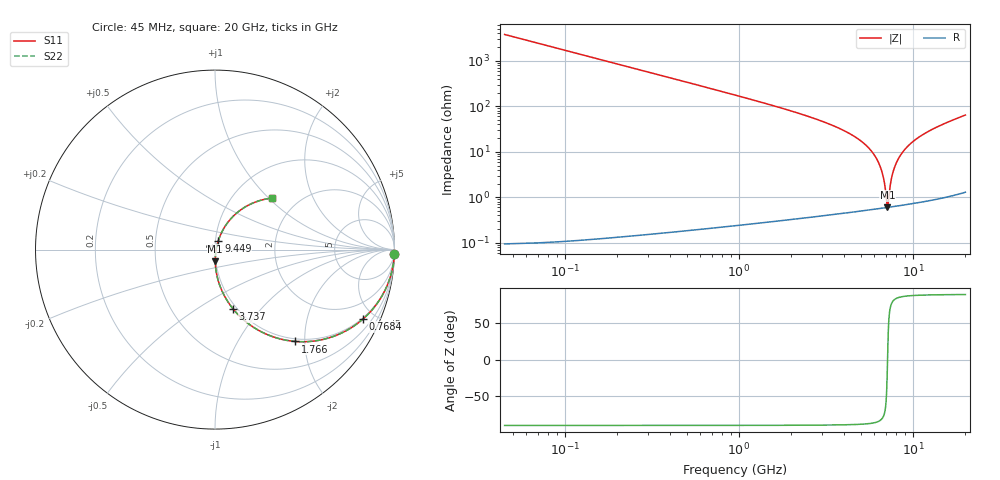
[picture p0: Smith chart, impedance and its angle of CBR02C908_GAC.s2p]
! S-parameter model data by Modelithics Inc.  support@modelithics.com 813-866-6335  Tampa FL USA
! S-Parameter data specifications:
! Substrate: 20-mil Rogers 4350B, substrate thickness, H=0.508mm, Dielectric constant, Er=3.75
! PCB Mounting Pad Footprint: Pad width, PadW=0.32mm , Pad length, PadL=0.37mm , Pad gap, PadG (edge-to-edge)=0.19mm , Reference planes=0.93mm apart
#  GHz  S  MA  R 50
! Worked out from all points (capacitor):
!   801 points, 45 MHz to 20 GHz, reference 50 ohm
!   read as one part in series: C = 929 fF near 144.8 MHz
!   lowest |Z| = 604 mohm at 7.129 GHz (marker M1)
!   series resonance near 7.139 GHz, so ESL is about 530 pH
!   S11 on the Smith chart (normalised r, x): 45 MHz: 1, -74; 768.4 MHz: 0.94, -4.29; 1.766 GHz: 0.95, -1.80; 3.737 GHz: 0.96, -0.72; 9.449 GHz: 1.03, +0.10; 20 GHz: 1.50, +1.05
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0.045  0.9997 -1.6  0.02626 88.4  0.02626 88.4  0.9997 -1.6
0.194662  0.9936 -6.7  0.113 83.3  0.113 83.3  0.9936 -6.7
0.319381  0.983 -10.9  0.1835 79.1  0.1835 79.1  0.983 -10.9
0.518931  0.9566 -17.5  0.2908 72.5  0.2908 72.5  0.9566 -17.5
0.768369  0.9108 -25.1  0.4119 64.8  0.4119 64.8  0.9108 -25.1
1.217356  0.8086 -37.2  0.5867 52.7  0.5867 52.7  0.8086 -37.2
1.766119  0.679 -48.9  0.7318 40.9  0.7318 40.9  0.679 -48.9
3.387462  0.3894 -70.1  0.9173 19.4  0.9173 19.4  0.3894 -70.1
3.736675  0.3446 -73.1  0.9347 16.2  0.9347 16.2  0.3446 -73.1
5.532625  0.1722 -84.2  0.9799 4.1  0.9799 4.1  0.1722 -84.2
6.704981  0.09132 -88.2  0.99 -1.8  0.99 -1.8  0.09132 -88.2
7.129025  0.0658 -88.6  0.9918 -3.7  0.9918 -3.7  0.0658 -88.6
7.802506  0.02851 -84.0  0.9932 -6.6  0.9932 -6.6  0.02851 -84.0
8.326325  0.006492 -13.8  0.9934 -8.7  0.9934 -8.7  0.006492 -13.8
8.4261  0.007877 25.2  0.9933 -9.1  0.9933 -9.1  0.007877 25.2
8.850144  0.02605 64.4  0.9928 -10.7  0.9928 -10.7  0.02605 64.4
9.448794  0.05354 69.6  0.9915 -13.0  0.9915 -13.0  0.05354 69.6
10.0225  0.07888 69.7  0.9895 -15.0  0.9895 -15.0  0.07888 69.7
11.39441  0.1357 67.0  0.9828 -19.7  0.9828 -19.7  0.1357 67.0
13.36496  0.2103 61.5  0.9688 -26.2  0.9688 -26.2  0.2103 61.5
16.68248  0.3246 51.8  0.9354 -36.5  0.9354 -36.5  0.3246 51.8
20  0.4301 41.9  0.8906 -46.5  0.8906 -46.5  0.4301 41.9
